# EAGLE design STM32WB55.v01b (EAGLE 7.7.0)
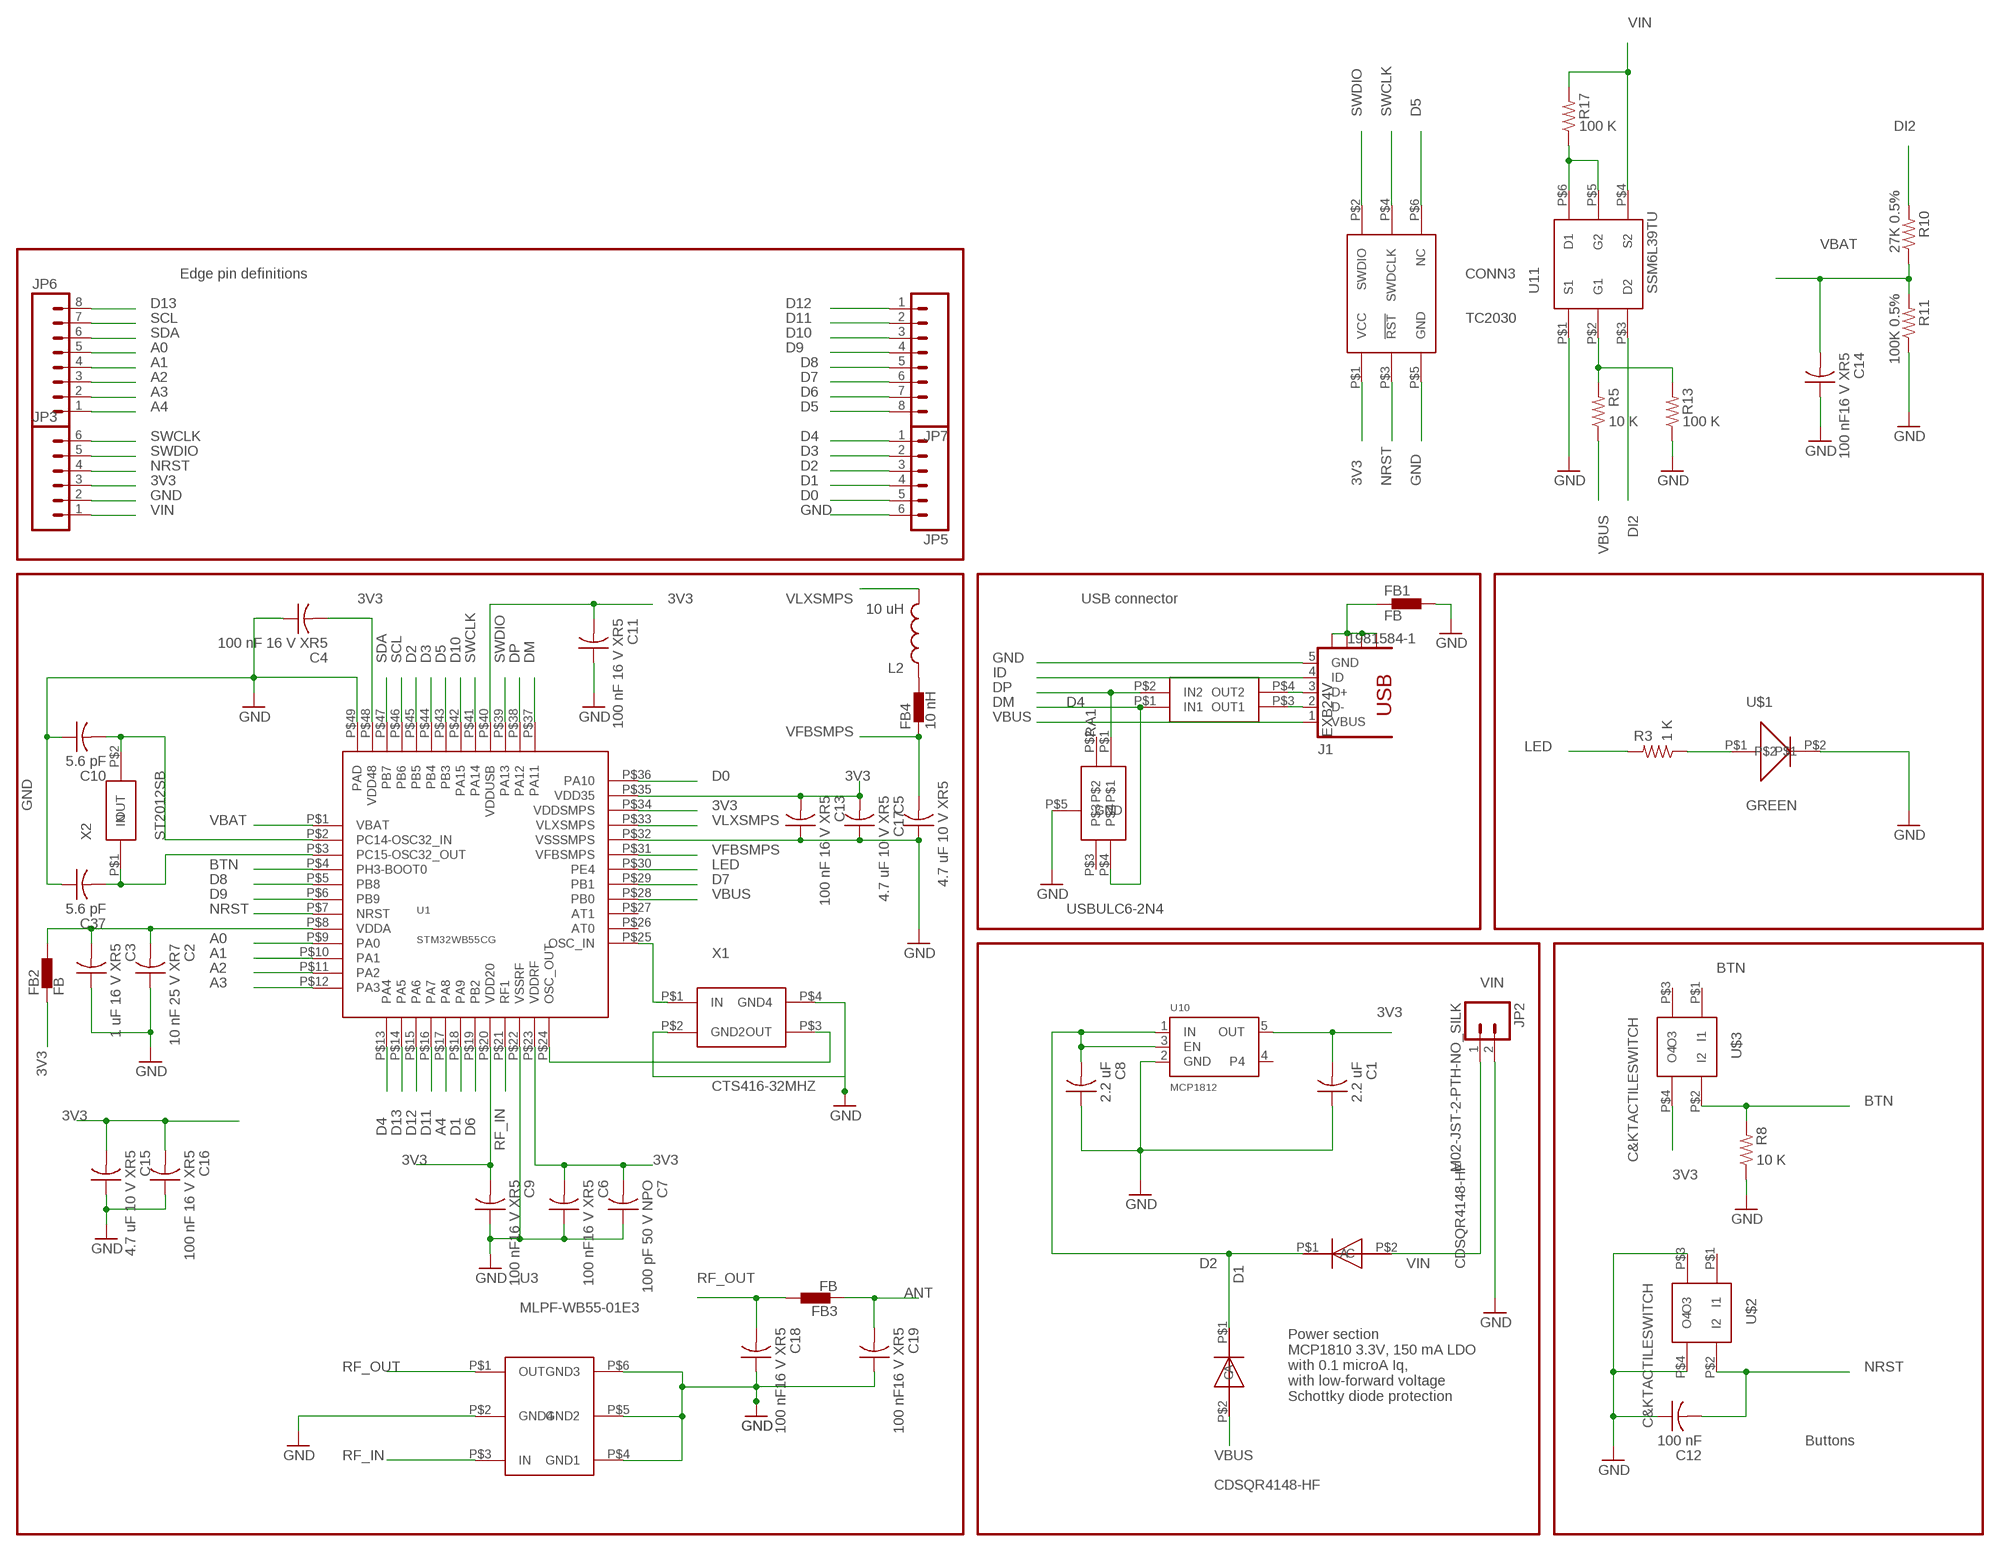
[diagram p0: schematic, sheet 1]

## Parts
C1  2.2 uF  C-US  [C0402_B]
C2  10 nF 25 V XR7  C-US  [C0402_B]
C3  1 uF 16 V XR5  C-US  [C0402_B]
C4  100 nF 16 V XR5  C-US  [C0402_B]
C5  4.7 uF 10 V XR5  C-US  [C0402_B]
C6  100 nF16 V XR5  C-US  [C0402_B]
C7  100 pF 50 V NPO  C-US  [C0402_B]
C8  2.2 uF  C-US  [C0402_B]
C9  100 nF16 V XR5  C-US  [C0402_B]
C10  5.6 pF  C-US  [C0402_B]
C11  100 nF 16 V XR5  C-US  [C0402_B]
C12  100 nF  C-US  [C0402_B]
C13  100 nF 16 V XR5  C-US  [C0402_B]
C14  100 nF16 V XR5  C-US  [C0402_B]
C15  4.7 uF 10 V XR5  C-US  [C0402_B]
C16  100 nF 16 V XR5  C-US  [C0402_B]
C17  4.7 uF 10 V XR5  C-US  [C0402_B]
C18  100 nF16 V XR5  C-US  [C0402_B]
C19  100 nF16 V XR5  C-US  [C0402_B]
C37  5.6 pF  C-US  [C0402_B]
CONN3  TC2030  [TC2030]
D1  CDSQR4148-HF  [CDSQR4148-HF]
D2  CDSQR4148-HF  [CDSQR4148-HF]
D4  USBULC6-2N4  [USBULC6-2N4]
FB1  FB  BLM15H  [0402]
FB2  FB  BLM15H  [0402]
FB3  FB  BLM15H  [0402]
FB4  10 nH  BLM15H  [0402]
J1  1981584-1  [1981584-1]
JP2  M02-JST-2-PTH-NO_SILK  [JST-2-PTH-NS]
JP3  M06NO_SILK  [1X06_NO_SILK]
JP5  M06NO_SILK  [1X06_NO_SILK]
JP6  M08NO_SILK  [1X08_NO_SILK]
JP7  M08NO_SILK  [1X08_NO_SILK]
L2  10 uH  INDUCTOR0805  [0805]
R3  1 K  R-US_  [R0402_B]
R5  10 K  R-US_  [R0402_B]
R8  10 K  R-US_  [R0402_B]
R10  27K 0.5%  R-US_  [R0402_B]
R11  100K 0.5%  R-US_  [R0402_B]
R13  100 K  R-US_  [R0402_B]
R17  100 K  R-US_  [R0402_B]
RA1  EXB24V  [EXB24V]
U1  STM32WB55CG  [ST32WB55CG]
U3  MLPF-WB55-01E3  [MLPF-WB55-01E3]
U10  MCP1812  VREG_SOT23-5  [SOT23-5]
U11  SSM6L39TU  [SSM6L39TU]
U$1  GREEN  0402LED  [0402LED]
U$2  C&KTACTILESWITCH  [C&KTACTILESWITCH]
U$3  C&KTACTILESWITCH  [C&KTACTILESWITCH]
X1  CTS416-32MHZ  [CTS416-32MHZ]
X2  ST2012SB  [ST2012SB]

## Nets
3V3: C1.2 C4.2 C5.2 C6.2 C7.2 C9.2 C11.2 C13.2 C15.2 C16.2 CONN3.P$1(VCC) FB2.1 JP3.3 U1.P$20(VDD20) U1.P$23(VDDRF) U1.P$34(VDDSMPS) U1.P$35(VDD35) U1.P$40(VDDUSB) U1.P$48(VDD48) U10.5(OUT) U$3.P$4(O4)
A0: JP6.5 U1.P$9(PA0)
A1: JP6.4 U1.P$10(PA1)
A2: JP6.3 U1.P$11(PA2)
A3: JP6.2 U1.P$12(PA3)
A4: JP6.1 U1.P$17(PA8)
ANT: C19.2 FB3.1
BTN: R8.2 U1.P$4(PH3-BOOT0) U$3.P$2(I2)
D0: JP5.5 U1.P$36(PA10)
D1: JP5.4 U1.P$18(PA9)
D2: JP5.3 U1.P$45(PB5)
D3: JP5.2 U1.P$44(PB4)
D4: JP5.1 U1.P$13(PA4)
D5: CONN3.P$6(NC) JP7.8 U1.P$43(PB3)
D6: JP7.7 U1.P$19(PB2)
D7: JP7.6 U1.P$29(PB1)
D8: JP7.5 U1.P$5(PB8)
D9: JP7.4 U1.P$6(PB9)
D10: JP7.3 U1.P$42(PA15)
D11: JP7.2 U1.P$16(PA7)
D12: JP7.1 U1.P$15(PA6)
D13: JP6.8 U1.P$14(PA5)
DI2: R10.2 U11.P$3(D2)
DM: D4.P$4 RA1.P$1(IN1) U1.P$37(PA11)
DP: D4.P$1 RA1.P$2(IN2) U1.P$38(PA12)
GND: C1.1 C2.1 C3.1 C4.1 C5.1 C6.1 C7.1 C8.1 C9.1 C10.1 C11.1 C12.1 C13.1 C14.1 C15.1 C16.1 C17.1 C18.1 C19.1 C37.1 CONN3.P$5(GND) D4.P$5(GND) FB1.2 J1.5(GND) JP2.2 JP3.2 JP5.6 R8.1 R11.1 R13.1 U1.P$22(VSSRF) U1.P$32(VSSSMPS) U1.P$49(PAD) U3.P$2(GND4) U3.P$4(GND1) U3.P$5(GND2) U3.P$6(GND3) U10.2(GND) U11.P$1(S1) U$1.P$2 U$2.P$3(O3) U$2.P$4(O4) X1.P$2(GND2) X1.P$4(GND4)
ID: J1.4(ID)
LED: R3.2 U1.P$30(PE4)
N$1: R3.1 U$1.P$1
N$2: C2.2 C3.2 FB2.2 U1.P$8(VDDA)
N$3: U1.P$25(OSC_IN) X1.P$1(IN)
N$4: U1.P$24(OSC_OUT) X1.P$3(OUT)
N$5: FB4.2 L2.1
N$7: C10.2 U1.P$2(PC14-OSC32_IN) X2.P$2(OUT)
N$8: C37.2 U1.P$3(PC15-OSC32_OUT) X2.P$1(IN)
N$12: R5.2 R13.2 U11.P$2(G1)
N$13: R17.1 U11.P$5(G2) U11.P$6(D1)
N$31: J1.3(D+) RA1.P$4(OUT2)
N$33: J1.2(D-) RA1.P$3(OUT1)
NRST: C12.2 CONN3.P$3(!RST) JP3.4 U1.P$7(NRST) U$2.P$2(I2)
PWRIN: C8.2 D1.P$1(C) D2.P$1(C) U10.1(IN) U10.3(EN)
RF_IN: U1.P$21(RF1) U3.P$3(IN)
RF_OUT: C18.2 FB3.2 U3.P$1(OUT)
SCL: JP6.7 U1.P$46(PB6)
SDA: JP6.6 U1.P$47(PB7)
SWCLK: CONN3.P$4(SWDCLK) JP3.6 U1.P$41(PA14)
SWDIO: CONN3.P$2(SWDIO) JP3.5 U1.P$39(PA13)
USB_SHIELD: FB1.1 J1.S1 J1.S2 J1.S3 J1.S4
VBAT: C14.2 R10.1 R11.2 U1.P$1(VBAT)
VBUS: D2.P$2(A) J1.1(VBUS) R5.1 U1.P$28(PB0)
VFBSMPS: C17.2 FB4.1 U1.P$31(VFBSMPS)
VIN: D1.P$2(A) JP2.1 JP3.1 R17.2 U11.P$4(S2)
VLXSMPS: L2.2 U1.P$33(VLXSMPS)
Unconnected: D4.P$2 D4.P$3 U1.P$26(AT0) U1.P$27(AT1) U10.4 U$2.P$1(I1) U$3.P$1(I1) U$3.P$3(O3)

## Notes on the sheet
- Edge pin definitions
- USB connector
- Power section
  MCP1810 3.3V, 150 mA LDO
  with 0.1 microA Iq, 
  with low-forward voltage 
  Schottky diode protection
- Buttons

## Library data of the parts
C1-C19 C37 = Spark:C-US: Capacitor
CONN3 = Kris:TC2030: TC2030 SWD pogo pin contact pad
D1 D2 = Kris:CDSQR4148-HF: ComChip's CDSQR4148-HF high speed 150 mA Io diode
D4 = Kris:USBULC6-2N4: ST TVS diode ESD Protection USBULC6-2N4
FB1-FB4 = STM32L433SARA.AssetTracker.v01:BLM15H: EMIFIL (R) Chip Ferrite Bead for GHz Noise
J1 = con-usb:1981584-1: Receptacle, micro-USB, type A/B Tyco Electronics; MF: Hirose; MPN: ZX62-AB-5PA(11)
JP2 = SparkFun-Connectors:M02: Standard 2-pin 0.1" header. Use with
JP3 JP5 = SparkFun-Connectors:M06: Header 6 Standard 6-pin 0.1" header. Use with straight break away headers (SKU : PRT-00116), right angle break away headers (PRT-00553), swiss pins (PRT-00743), machine pins (PRT-00117), and female headers (PRT-00115). Molex polarized connector foot print use with SKU : PRT-08094 with associated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
JP6 JP7 = SparkFun-Connectors:M08: Header 8 Standard 8-pin 0.1" header. Use with straight break away headers (SKU : PRT-00116), right angle break away headers (PRT-00553), swiss pins (PRT-00743), machine pins (PRT-00117), and female headers (PRT-00115).
L2 = SparkFun-Passives:INDUCTOR: Inductors
R3 R5 R8 R10 R11 R13 R17 = Spark:R-US_: 0402 Resistor
RA1 = Kris:EXB24V: Panasonic EXB24 22 Ohm series resistor pair
U1 = Kris:STM32WB55CG: STM32WB55CG 7 mm x 7 mm UFQFPN48 https://www.st.com/en/microcontrollers/stm32wbx5.html?querycriteria=productId=LN2047
U3 = Kris:MLPF-WB55-01E3: MLPF-WB55-01E3
U10 = ModernDevice:VREG_SOT23-5: SOT23-5 Fixed Voltage Regulators To better organise some of the SOT23-5 fixed voltage regulators in this library, this new part was created. Part Current Out V Out V In V Dropout Digikey Part No. ADP121 150mA 3.3V 3.4-5.5V 0.09V @ 150mA ADP121-AUJZ33R7CT-ND ADP121 150mA 3.0V 3.1-5.5V 0.09V @ 150mA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
U11 = Kris:SSM6L39TU: SSM6L39TU Dual Mosfet https://www.mouser.com/datasheet/2/408/SSM6L39TU_datasheet_en_20140301-771389.pdf
U$1 = Kris:0402LED: 0402led
U$2 U$3 = Kris:C&KTACTILESWITCH: C&K Tactile Switch 611-PTS810SJS250SMTR
X1 = Kris:CTS416-32MHZ: 32 MHz CTS416 crystal
X2 = Kris:ST2012SB: Kyocera 2.0 x 1.2 mm 32.768 20kHz ppm 4 pf crystal

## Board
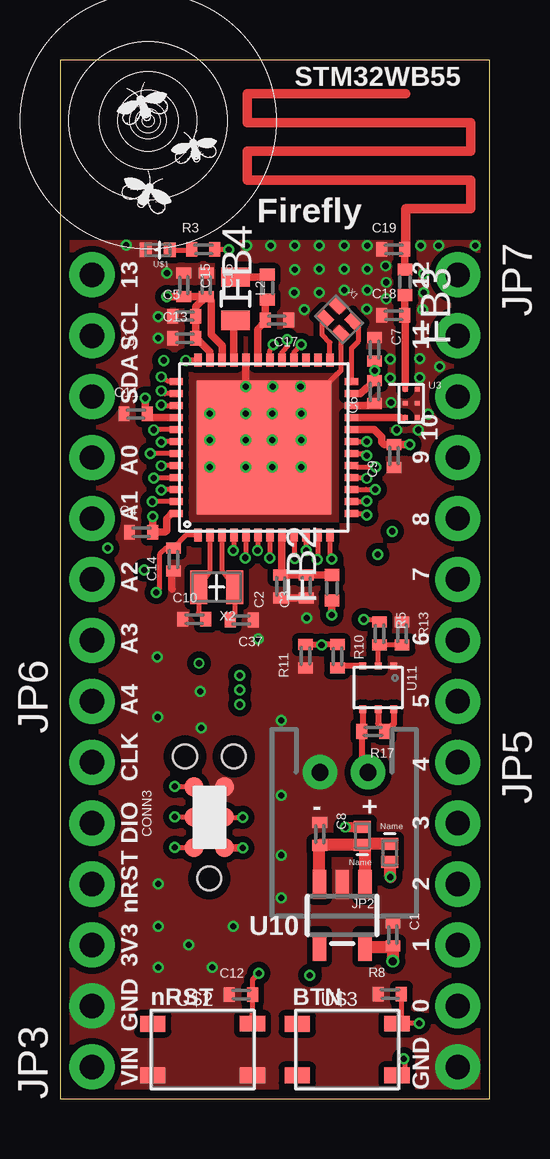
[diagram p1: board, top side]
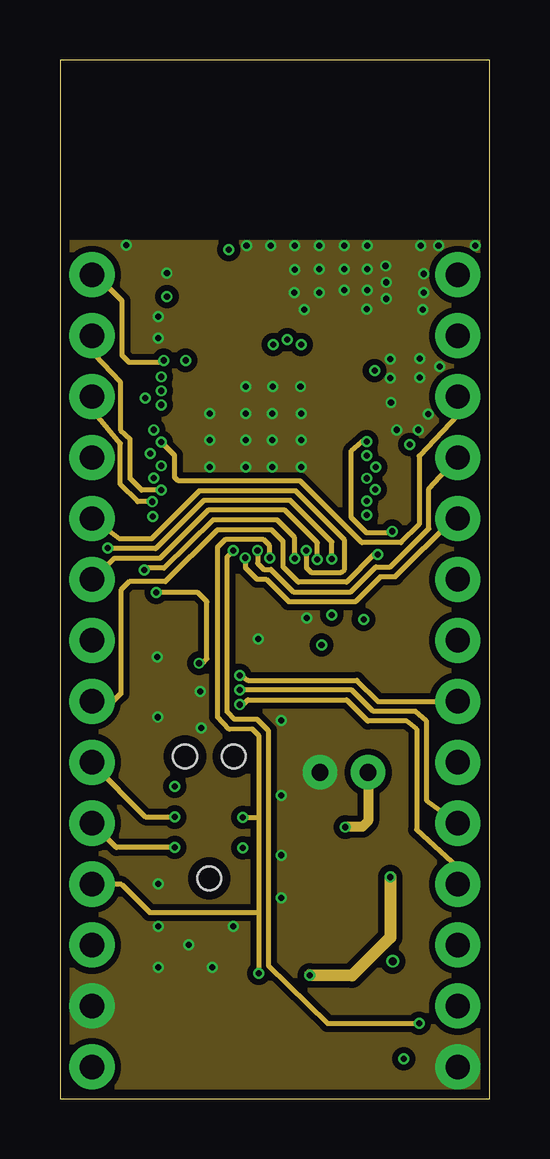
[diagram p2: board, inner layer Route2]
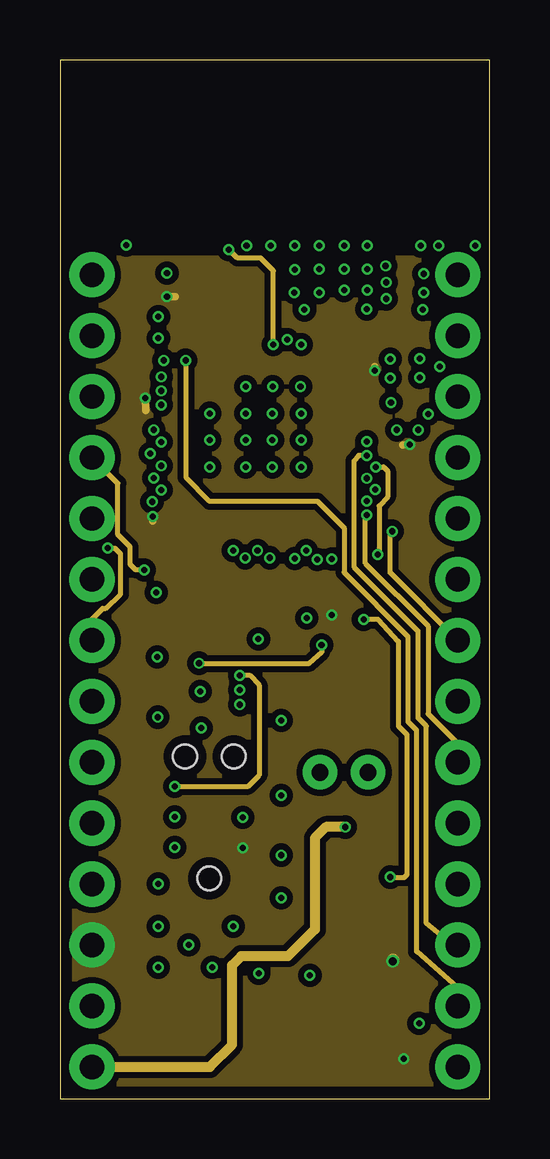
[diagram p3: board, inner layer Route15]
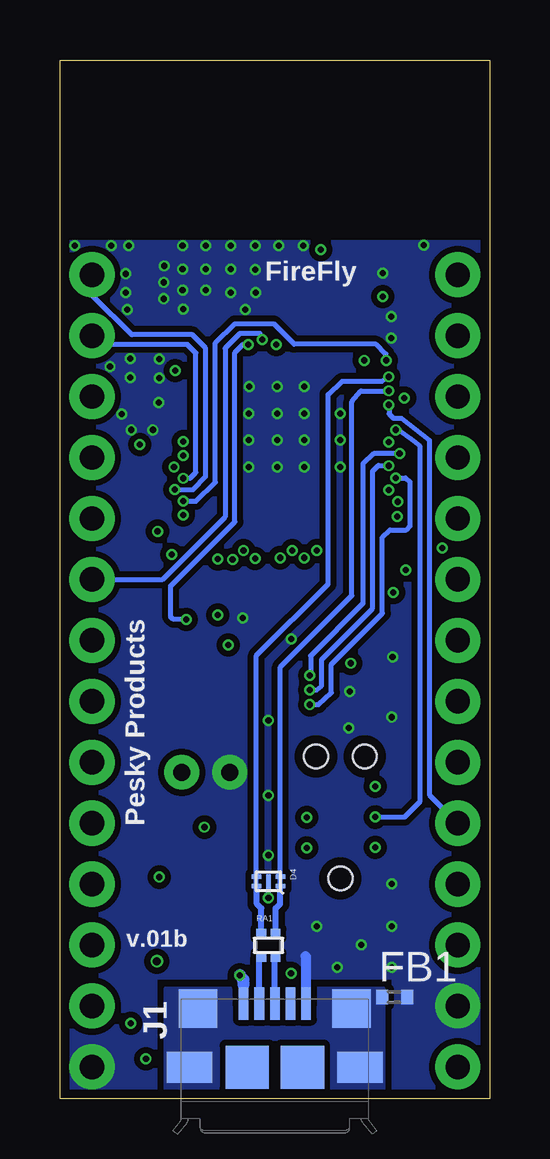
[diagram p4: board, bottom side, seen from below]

Size 17.91 x 43.31 mm. Coordinates in mm from the lower left corner, seen from the top.
Outline: 0,0 17.91,0 17.91,43.31 0,43.31 0,0
Copper layers (1*2*15*16): Top 0.035559375mm / dielectric 0.17018125mm / Route2 0.01778125mm / dielectric 47mil / Route15 0.01778125mm / dielectric 0.17018125mm / Bottom 0.035559375mm
Design rules "OSHPark-4layer *": minimum track width 5mil, minimum drill 10mil, track to track 5mil, track to pad 5mil, pad to pad 5mil, via to via 5mil, smd to smd 5mil, copper to edge 15mil, drill to drill 6mil, minimum pad ring 4mil, minimum via ring 4mil, stop-mask expansion 4mil, vias tented up to drill 20mil, thermal gap 10mil

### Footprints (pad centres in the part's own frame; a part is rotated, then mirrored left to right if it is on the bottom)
C0402_B = smd 0.457 x 0.61: 1 -0.483,0; 2 0.483,0
TC2030 = smd 0.787 x 0.787: P$1 -1.27,-0.635; P$2 -1.27,0.635; P$3 0,-0.635; P$4 0,0.635; P$5 1.27,-0.635; P$6 1.27,0.635 | hole 0.991: -2.54,0; 2.54,1.016; 2.54,-1.016
CDSQR4148-HF = smd 0.7 x 0.5: P$1 0,0.375; P$2 0,-0.375
USBULC6-2N4 = smd 0.2 x 0.4: P$1 0.2,0.5; P$2 -0.2,0.5; P$3 -0.2,-0.5; P$4 0.2,-0.5 | smd 0.6 x 0.2: P$5 0,0
0402 = smd 0.5 x 0.61: 1 -0.5,0; 2 0.55,0
1981584-1 = smd 0.4 x 1.35: 1 -1.3,4.1; 2 -0.65,4.1; 3 0,4.1; 4 0.65,4.1; 5 1.3,4.1 | smd 1.8 x 1.8: M1 -1.15,1.45; M2 1.15,1.45 | smd 1.9 x 1.3: S1 -3.55,1.45; S2 3.55,1.45 | smd 1.6 x 1.6: S3 -3.2,3.885; S4 3.2,3.885
JST-2-PTH-NS = drill 0.7 pad 1.448: 1 -1,0; 2 1,0
1X06_NO_SILK = drill 1.016 pad 1.88: 1 0,0; 2 2.54,0; 3 5.08,0; 4 7.62,0; 5 10.16,0; 6 12.7,0
1X08_NO_SILK = drill 1.016 pad 1.88: 1 0,0; 2 2.54,0; 3 5.08,0; 4 7.62,0; 5 10.16,0; 6 12.7,0; 7 15.24,0; 8 17.78,0
0805 = smd 0.8 x 1.2: 1 -0.9,0; 2 0.9,0
R0402_B = smd 0.457 x 0.61: 1 -0.483,0; 2 0.483,0
EXB24V = smd 0.4 x 0.36: P$1 -0.3,0.5; P$2 0.3,0.5; P$3 -0.3,-0.5; P$4 0.3,-0.5
ST32WB55CG = smd 0.55 x 0.3: P$1 -3.65,2.75; P$2 -3.65,2.25; P$3 -3.65,1.75; P$4 -3.65,1.25; P$5 -3.65,0.75; P$6 -3.65,0.25; P$7 -3.65,-0.25; P$8 -3.65,-0.75; P$9 -3.65,-1.25; P$10 -3.65,-1.75; P$11 -3.65,-2.25; P$12 -3.65,-2.75; P$25 3.65,-2.75; P$26 3.65,-2.25; P$27 3.65,-1.75; P$28 3.65,-1.25; P$29 3.65,-0.75; P$30 3.65,-0.25; P$31 3.65,0.25; P$32 3.65,0.75; P$33 3.65,1.25; P$34 3.65,1.75; P$35 3.65,2.25; P$36 3.65,2.75 | smd 0.3 x 0.55: P$13 -2.75,-3.65; P$14 -2.25,-3.65; P$15 -1.75,-3.65; P$16 -1.25,-3.65; P$17 -0.75,-3.65; P$18 -0.25,-3.65; P$19 0.25,-3.65; P$20 0.75,-3.65; P$21 1.25,-3.65; P$22 1.75,-3.65; P$23 2.25,-3.65; P$24 2.75,-3.65; P$37 2.75,3.65; P$38 2.25,3.65; P$39 1.75,3.65; P$40 1.25,3.65; P$41 0.75,3.65; P$42 0.25,3.65; P$43 -0.25,3.65; P$44 -0.75,3.65; P$45 -1.25,3.65; P$46 -1.75,3.65; P$47 -2.25,3.65; P$48 -2.75,3.65 | smd 5.6 x 5.6: P$49 0,0
MLPF-WB55-01E3 = smd 0.2 x 0.2: P$1 -0.25,0.587; P$2 -0.25,0; P$3 -0.25,-0.587; P$4 0.25,-0.587; P$5 0.25,0; P$6 0.25,0.587
SOT23-5 = smd 0.55 x 1.2: 1 -0.95,-1.3; 2 0,-1.3; 3 0.95,-1.3; 4 0.95,1.3; 5 -0.95,1.3
SSM6L39TU = smd 0.3 x 0.3: P$1 -0.9,0.65; P$2 -0.9,0; P$3 -0.9,-0.65; P$4 0.9,-0.65; P$5 0.9,0; P$6 0.9,0.65
0402LED = smd 0.5 x 0.6: P$1 -0.5,0; P$2 0.5,0
C&KTACTILESWITCH = smd 1.05 x 0.65: P$1 -2.075,1.073; P$2 2.075,1.075; P$3 -2.075,-1.075; P$4 2.075,-1.075
CTS416-32MHZ = smd 0.67 x 0.48: P$1 -0.485,-0.38; P$2 0.485,-0.38; P$3 0.485,0.38; P$4 -0.485,0.38
ST2012SB = smd 0.7 x 1.4: P$1 -0.75,0; P$2 0.75,0

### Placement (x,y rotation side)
C1  13.87,6.86 270 top
C2  9.19,21.36 90 top
C3  10.26,21.36 90 top
C4  3.38,23.62 0 top
C5  5.18,32.63 0 top
C6  13.11,29.46 90 top
C7  13.11,31.24 270 top
C8  10.82,11.05 270 top
C9  13.92,26.8 90 top
C10  5.59,19.99 0 top
C11  3.15,28.55 0 top
C12  7.54,4.34 0 top
C13  5.18,31.7 0 top
C14  4.72,22.48 90 top
C15  5.16,33.93 270 top
C16  6.1,33.93 270 top
C17  9.04,32.46 180 top
C18  13.89,32.66 0 top
C19  13.89,35.41 0 top
C37  7.57,19.96 180 top
CONN3  6.22,11.73 90 top
D1  12.6,10.97 180 top
D2  13.74,10.26 0 top
D4  9.22,9.07 270 bottom
FB1  3.99,4.24 0 bottom
FB2  11.33,21.29 90 top
FB3  14.37,34.06 270 top
FB4  8.64,33.81 90 top
J1  8.95,-0.13 0 bottom
JP2  11.84,13.61 180 top
JP3  1.33,1.33 90 top
JP5  16.57,14.03 270 top
JP6  1.33,16.57 90 top
JP7  16.57,34.35 270 top
L2  7.32,33.35 270 top
R3  5.97,35.41 0 top
R5  13.31,19.41 270 top
R8  13.74,4.37 0 top
R10  11.56,18.45 270 top
R11  10.22,18.45 90 top
R13  14.25,19.41 270 top
R17  13.06,15.32 180 top
RA1  9.22,6.4 0 bottom
U1  8.5,27.15 90 top
U3  14.63,28.99 0 top
U10  11.76,7.65 180 top
U11  13.26,17.14 270 top
U$1  4.06,35.38 180 top
U$2  5.94,2.06 0 top
U$3  11.96,2.06 0 top
X1  11.63,32.49 315 top
X2  6.53,21.34 180 top

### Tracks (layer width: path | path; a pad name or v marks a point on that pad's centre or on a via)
3V3  (via drill 0.25, 0.33)
  Top 0.203: U$3.P$4 14.38,1.22 14.38,1.63 v14.33,1.68
  Top 0.305: U1.P$35 6.25,31.14 5.69,31.7 5.69,31.67 C13.2 C5.2 5.66,33.03 C16.2 | U1.P$40 3.62,28.4 3.68,28.42 3.68,28.43 | C7.2 v13.11,30.35 C6.2 12.51,29.4 U1.P$23 | v3.86,24.28 C4.2 4.37,23.62 4.45,23.7 4.45,24.18 4.64,24.4 U1.P$48 | v14.58,27.28 C9.2 13.51,27.28 13.41,27.38 13.41,27.58 13.09,27.9 U1.P$20 | 3.68,28.43 C11.2 3.56,28.7 v3.56,29.21 | 3.68,28.43 3.68,28.46 | 11.37,20.84 FB2.1 v11.33,20.17 | C16.2 6.12,33.4 6.3,33.27 6.3,31.85 6.76,31.39 6.76,30.81 U1.P$34 | C16.2 C15.2 4.45,33.45 v4.46,33.44 | CONN3.P$1 v7.62,10.46
  Top 0.508: U10.5 13.86,6.34 | 13.86,6.34 C1.2 | 13.86,6.34 13.86,5.77 v13.87,5.74
  Route15 0.203: v14.33,1.68 14.33,1.63 14.38,1.57
  Route15 0.305: v3.56,29.21 3.58,28.69 | v13.11,30.35 13.11,30.53 | v3.86,24.28 3.86,24.08 | v14.58,27.28 14.28,27.25 | v4.46,33.44 4.8,33.44 | v11.33,20.17 11.33,20.24
  Route15 0.508: v13.87,5.74 13.89,5.79 13.87,5.82
  pour Route15 (isolate 0.254, no thermals): 0.64,35.05 17.27,35.05 17.27,0.64 0.64,0.64
A0  (via drill 0.25)
  Top 0.203: v9.78,22.53 9.78,23.41 U1.P$9
  Route2 0.203: v9.78,22.53 9.78,23.39 9.04,24.13 6.38,24.13 4.34,22.12 3.5,22.12 v3.5,22.05
  Route15 0.203: v3.5,22.05 3.15,22.05 2.92,22.28 2.92,23.01 2.41,23.52 2.41,25.65 JP6.5
A1  (via drill 0.25)
  Top 0.203: U1.P$10 10.25,22.88 v10.26,22.86
  Route2 0.203: JP6.4 2.49,23.34 3.81,23.34 5.82,25.35 9.8,25.35 11.86,23.29 11.86,22.07 11.71,21.95 10.46,21.95 10.26,22.15 v10.26,22.86
A2  (via drill 0.25)
  Top 0.203: U1.P$11 10.75,22.58 v10.72,22.48
  Route2 0.203: v10.72,22.48 10.72,23.19 9.37,24.54 6.17,24.54 4.17,22.53 2.26,22.53 JP6.3
A3  (via drill 0.25)
  Top 0.203: U1.P$12 11.25,22.69 v11.33,22.5
  Route2 0.203: v11.33,22.5 11.33,23.22 9.6,24.94 5.99,24.94 3.99,22.94 2.08,22.94 v1.98,22.96
  Route15 0.203: v1.98,22.96 2.29,22.96 2.52,22.73 2.52,21.03 1.91,20.45 1.78,20.45 1.33,20 JP6.2
A4  (via drill 0.25)
  Top 0.203: U1.P$17 12.33,26.4 12.37,26.34 v13.16,26.34
  Route2 0.203: JP6.1 1.35,16.59 2.21,16.59 2.54,16.89 2.54,21.21 2.9,21.57 4.39,21.57 6.55,23.72 8.81,23.72 9.3,23.24 9.3,22.17 9.93,21.54 11.94,21.54 13.08,22.68 v13.25,22.7
  Route15 0.203: v13.16,26.34 13.49,26.34 13.65,26.18 13.65,25.09 13.3,24.71 13.3,22.75 v13.25,22.7
ANT
  Top 0.305: FB3.1 C19.2 14.38,35.41 14.41,35.43
  Top 0.4: 14.41,35.43 14.41,37.1 17.11,37.1 17.11,38.3 7.81,38.3 7.81,39.5 17.11,39.5 17.11,40.7 7.81,40.7 7.81,41.9 14.41,41.9
BTN  (via drill 0.25)
  Top 0.203: U1.P$4 7.25,22.94 v7.21,22.86 | v14.96,3.15 13.98,3.15 U$3.P$2 14.22,3.39 R8.2
  Route2 0.203: v14.96,3.15 11.15,3.15 8.69,5.56 8.69,15.35 8.22,15.82 7.28,15.82 6.96,16.14 6.96,22.58 v7.21,22.86
D0  (via drill 0.25)
  Top 0.203: U1.P$36 5.33,30.8 v5.23,30.79
  Route15 0.203: JP5.5 16.57,4.64 14.86,6.15 14.86,15.37 14.5,15.72 14.5,19.25 11.84,21.95 11.84,23.8 10.72,24.92 6.22,24.92 5.26,25.91 5.26,30.76 v5.23,30.79
D1  (via drill 0.25)
  Top 0.203: U1.P$18 12.62,26.9 v12.78,26.81
  Route15 0.203: JP5.4 16.34,6.41 15.27,7.32 15.27,15.54 14.91,15.9 14.91,19.51 12.24,22.17 12.24,26.59 12.45,26.82 v12.78,26.81
D2  (via drill 0.25)
  Top 0.203: U1.P$45 4.7,25.9 4.67,25.93 4.7,25.93 4.62,25.88 v3.91,25.88
  Route2 0.203: JP5.3 16.59,8.97 16.59,9.65 14.86,11.23 14.86,15.42 14.45,15.75 12.83,15.75 11.94,16.64 7.82,16.64 7.64,16.43 v7.49,16.43
  Bottom 0.203: v3.91,25.88 3.5,25.88 3.33,25.73 3.33,23.88 3.48,23.72 4.17,23.72 4.47,23.42 4.47,20.24 6.6,18.11 6.6,16.94 7.14,16.43 v7.49,16.43
D3  (via drill 0.25)
  Top 0.203: U1.P$44 4.25,26.4 v4.22,26.39
  Route2 0.203: v7.49,17.04 12.17,17.04 13.06,16.15 14.81,16.15 15.27,15.75 15.27,12.45 JP5.2
  Bottom 0.203: v4.22,26.39 4.31,26.4 4.64,26.4 4.88,26.17 4.88,20.45 7.01,18.31 7.01,17.22 7.21,17.04 v7.49,17.04
D4  (via drill 0.25)
  Top 0.203: U1.P$13 12.68,24.4 v12.78,24.33
  Route15 0.203: v12.78,24.33 12.72,24.16 12.72,22.33 15.34,19.71 15.34,16.05 16.57,14.82 JP5.1
D5  (via drill 0.25)
  Top 0.203: U1.P$43 v3.76,26.9 | CONN3.P$6 4.78,13.01 v4.78,13.03
  Route2 0.203: JP7.8 13.26,16.56 12.37,17.45 7.82,17.45 7.57,17.65 v7.49,17.65
  Route15 0.203: 7.48,17.67 7.52,17.67 | 7.52,17.67 7.9,17.67 8.29,17.25 8.29,13.49 7.84,13.03 v4.78,13.03 | v7.49,17.65 7.51,17.65 7.52,17.67
  Bottom 0.203: v3.76,26.9 4.83,26.9 5.28,26.47 5.28,20.65 7.47,18.47 7.47,17.7 v7.49,17.65
D6  (via drill 0.25)
  Top 0.203: U1.P$19 12.72,27.4 v12.78,27.39
  Route2 0.203: v13.84,23.66 13.6,23.6 12.78,23.6 12.14,24.23 12.14,27.03 12.57,27.41 12.76,27.41 v12.78,27.39
  Route15 0.203: JP7.7 13.75,21.93 13.75,23.66 v13.84,23.66
D7  (via drill 0.25)
  Top 0.203: U1.P$29 9.25,31.09 9.47,31.37 v9.47,31.65
  Bottom 0.203: v9.47,31.65 9.47,31.77 9.58,31.9 10.41,31.9 11.02,31.29 11.02,24.26 13.63,21.65 JP7.6
D8  (via drill 0.25)
  Top 0.203: U1.P$5 7.75,22.61 v7.72,22.55
  Route2 0.203: v7.72,22.55 7.72,22.15 8.2,21.67 8.59,21.67 9.53,20.73 12.32,20.73 13.36,21.77 13.97,21.77 16.38,24.18 JP7.5
D9  (via drill 0.25)
  Top 0.203: U1.P$6 8.25,22.98 v8.23,22.86
  Route2 0.203: JP7.4 15.37,25.43 15.37,23.77 13.77,22.17 13.16,22.17 12.12,21.13 9.73,21.13 8.79,22.07 8.48,22.07 8.23,22.33 v8.23,22.86
D10  (via drill 0.25)
  Top 0.203: U1.P$42 4.42,27.4 v4.22,27.38
  Route2 0.203: JP7.3 16.57,28.51 14.96,26.8 14.96,23.95 14.2,23.19 12.57,23.19 10.01,25.76 4.93,25.76 4.78,25.91 4.78,26.82 v4.22,27.38
D11  (via drill 0.25)
  Top 0.203: U1.P$16 12.71,25.9 v12.78,25.87
  Bottom 0.203: v12.78,25.87 12.48,25.87 12.24,26.11 12.24,31.09 12.6,31.45 16.15,31.45 JP7.2
D12  (via drill 0.25)
  Top 0.203: U1.P$15 12.75,25.4 v13.13,25.4
  Bottom 0.203: v13.13,25.4 12.36,25.4 11.84,25.93 11.84,31.29 12.39,31.85 14.91,31.85 16.57,33.49 JP7.1
D13  (via drill 0.25)
  Top 0.203: U1.P$14 12.66,24.9 v12.78,24.92
  Route2 0.203: JP6.8 1.5,34.35 2.58,33.27 2.58,31 2.87,30.71 4.24,30.71 v4.32,30.79
  Bottom 0.203: v12.78,24.92 12.24,24.92 11.43,25.7 11.43,31.52 10.62,32.31 9,32.31 8.15,31.46 4.74,31.46 4.33,31.05 4.33,30.79 v4.32,30.79
DI2
  Top 0.254: U11.P$3 11.63,18.05 R10.2
DM  (via drill 0.25)
  Top 0.203: U1.P$37 4.51,29.9 v4.22,30.1
  Bottom 0.203: D4.P$4 9.72,18.47 6.73,21.46 6.73,29.36 6.15,29.92 4.48,29.92 v4.22,30.1
  Bottom 0.254: RA1.P$1 9.52,7.95 9.7,8.13 9.7,8.85 D4.P$4
DP  (via drill 0.25)
  Top 0.203: U1.P$38 4.37,29.4 v4.22,29.52
  Bottom 0.203: D4.P$1 8.72,18 5.74,20.98 5.74,29.06 5.37,29.52 v4.22,29.52
  Bottom 0.254: RA1.P$2 8.92,7.95 8.74,8.13 8.74,8.85 D4.P$1
GND  (via drill 0.25)
  Top 0.203: X1.P$2 11.71,30.35 v8.85,27.46
  Top 0.305: U1.P$32 7.75,29.95 7.75,30.02 | U1.P$22 13.08,28.9 C6.1 | C14.1 4.65,22.05 4.65,21.29 4.67,21.26 | C2.1 C3.1
  Bottom 0.203: D4.P$5 v9.22,8.38
  Bottom 0.406: J1.5 7.65,5.93 7.67,5.94
  other vias: 7.73,27.46 11.84,35.56 15.04,35.56 15.16,33.6 13.59,33.35 12.8,33.71 12.8,35.56 15.11,32.89 13.77,30.84 14.99,30.86 14.99,30.07 13.77,30.05 13.79,29.03 9.22,10.16 9.22,12.65 6.24,28.57 8.85,26.34 7.73,29.69 8.85,28.57 7.73,28.57 7.73,26.34 6.24,26.34 6.24,27.46 12.78,32.92 2.76,35.59 4.46,34.42 4.1,32.6 15.34,28.55 15.82,30.53 14.94,27.89 10.79,35.56 9.78,35.56 8.79,35.56 7.77,35.56 11.84,34.59 10.79,34.59 11.84,33.71 17.3,35.56 15.77,35.56 15.16,34.39 10.05,28.57 10.05,27.46 10.05,26.34 8.27,19.18 9.22,15.77 10.29,20.05 4.1,31.71 9.78,34.57 10.79,33.6 9.75,33.6 10.19,32.89 14.03,27.89 4.05,18.43 4.08,15.91 5.84,16.98 5.88,15.46 10.02,29.69 8.86,29.69 13.56,34.72 12.8,34.59 13.59,34.04 4.09,7.19 6.35,5.49 7.21,7.19 4.09,5.49 5.36,6.43 4.09,8.97
  pour Route2 (isolate 0.254, no thermals): 0,35.69 17.91,35.69 17.91,0 0,0
  pour Top (isolate 0.254, no thermals): 0,35.69 17.91,35.69 17.91,0 0,0
  pour Bottom (isolate 0.254, no thermals): 13.97,0 17.91,0 17.91,35.69 0,35.69 0,0 3.96,0 3.96,5.08 13.97,5.08
LED  (via drill 0.25)
  Top 0.203: U1.P$30 8.75,31.2 v8.89,31.45 | v7.04,35.41 R3.2
  Route15 0.203: v8.89,31.45 8.89,34.52 8.36,35.05 7.39,35.05 v7.04,35.41
N$1
  Top 0.203: U$1.P$1 5.46,35.38 R3.1
N$2
  Top 0.305: U1.P$8 9.25,21.95 C2.2 C3.2 FB2.2
N$3
  Top 0.203: U1.P$25 11.25,31.53 10.92,31.85 10.92,32.54 X1.P$1
N$4
  Top 0.203: U1.P$24 12.15,31.3 12.45,31.6 12.45,32.29 X1.P$3
N$5
  Top 0.305: L2.1 8.52,34.25 FB4.2
N$7
  Top 0.203: U1.P$2 6.25,21.96 X2.P$2 5.78,20.28 C10.2
N$8
  Top 0.203: U1.P$3 6.75,22.02 X2.P$1 7.28,20.21 C37.2
N$12
  Top 0.203: R13.2 R5.2 13.26,19 U11.P$2
N$13
  Top 0.254: U11.P$5 13.26,15.65 R17.1 13.91,15.64 U11.P$6
N$31
  Bottom 0.254: J1.3 8.95,5.87 RA1.P$4
N$33
  Bottom 0.254: J1.2 9.6,5.82 RA1.P$3
NRST  (via drill 0.25)
  Top 0.203: U$2.P$2 C12.2 8.03,4.98 v8.28,5.23 | U1.P$7 8.75,22.67 v8.74,22.55 | CONN3.P$3 v7.62,11.73
  Route2 0.203: v8.74,22.55 8.74,23.06 8.48,23.32 6.88,23.32 6.55,22.99 6.55,15.94 7.06,15.4 8.01,15.42 8.28,15.15 8.28,11.73 | 8.28,11.73 8.28,7.8 | 8.28,7.8 v8.28,5.23 8.27,5.22 | JP3.4 1.35,8.94 2.56,8.94 3.73,7.77 8.26,7.77 8.28,7.8 | v7.62,11.73 8.28,11.73
PWRIN
  Top 0.406: 12.97,10.64 D1.P$1 12.71,10.49 | 10.85,10.6 C8.2
  Top 0.508: D2.P$1 12.97,10.64 | D1.P$1 10.85,10.6 | U10.3 10.81,10.56 C8.2 | U10.1 12.71,10.49
RF_IN
  Top 0.203: U3.P$3
  Top 0.254: 14.18,28.4 U3.P$3
  Top 0.305: U1.P$21 14.18,28.4
RF_OUT
  Top 0.254: U3.P$1 14.38,29.57 14.38,29.77
  Top 0.305: 14.38,29.77 C18.2 FB3.2
SCL  (via drill 0.25)
  Top 0.203: U1.P$46 4.24,25.4 v4.22,25.38
  Route2 0.203: JP6.7 1.44,31.71 1.44,31.03 2.52,29.87 2.52,27.89 2.92,27.51 2.92,25.86 3.4,25.38 v4.22,25.38
SDA  (via drill 0.25)
  Top 0.203: U1.P$47 3.83,24.9 v3.83,24.89
  Route2 0.203: v3.83,24.89 3.23,24.89 2.52,25.61 2.52,27.33 1.52,28.52 1.52,29.09 JP6.6
SWCLK  (via drill 0.25)
  Top 0.203: 4.81,27.94 U1.P$41 4.08,27.9 v3.91,27.89 | CONN3.P$4 5.08,11.73 v4.78,11.75
  Route2 0.203: JP3.6 1.33,13.98 3.56,11.76 4.76,11.76 v4.78,11.75
  Bottom 0.203: v3.91,27.89 3.79,27.89 3.28,27.51 2.92,27.23 2.92,12.37 3.56,11.73 4.76,11.73 v4.78,11.75
SWDIO  (via drill 0.25)
  Top 0.203: v4.22,28.93 4.29,28.91 U1.P$39 | CONN3.P$2 5,10.46 v4.78,10.48
  Route2 0.203: v4.78,10.48 2.35,10.48 JP3.5
  Bottom 0.203: JP3.5 2.52,12.68 2.52,27.46 3.68,28.37 4.01,28.37 4.19,28.55 4.19,28.88 v4.22,28.93
USB_SHIELD
  pour Bottom (isolate 0.254, no thermals): 4.47,0 13.46,0 13.46,4.57 4.47,4.57
VBAT  (via drill 0.25)
  Top 0.203: U1.P$1 5.24,23.5 C14.2 4.42,22.96 4.14,22.68 4.14,21.26 v4.01,21.11
  Top 0.254: R11.2 10.88,18.94 v10.9,18.92 11.04,18.94 R10.1
  Route2 0.203: v5.79,18.16 5.94,18.16 6.12,18.34 6.12,20.73 5.74,21.11 v4.01,21.11
  Route15 0.203: v5.79,18.16 10.39,18.16 10.9,18.62 v10.9,18.92
VBUS  (via drill 0.25)
  Top 0.203: U1.P$28 9.75,31.11 v10.06,31.45 | v12.65,19.99 13.13,19.99 R5.1
  Top 0.406: 13.77,9.86 D2.P$2
  Top 0.508: v13.77,9.25 13.77,9.86
  Route2 0.508: v13.77,9.25 13.77,6.73 12.17,5.13 v10.41,5.16
  Route15 0.203: 13.72,9.3 v13.77,9.25 13.79,9.22 14.33,9.22 14.45,9.35 14.45,15.19 14.1,15.54 14.1,19.07 13.26,19.99 v12.65,19.99
  Bottom 0.203: v10.06,31.45 10.29,31.45 10.62,31.11 10.62,24.05 13.31,21.36 13.31,20.12 13.18,19.99 v12.65,19.99
  Bottom 0.406: J1.1 10.25,4.77
  Bottom 0.508: 10.25,4.77 10.26,4.98 v10.41,5.16
VFBSMPS
  Top 0.305: U1.P$31 8.25,32.07 C17.2 8.56,33.23 FB4.1
VIN  (via drill 0.25)
  Top 0.254: U11.P$4 12.61,15.33 R17.2 12.57,13.88 JP2.1
  Top 0.406: v11.89,11.33 12.41,11.33 D1.P$2
  Route2 0.406: JP2.1 12.84,11.59 D1.P$2 11.91,11.35 v11.89,11.33
  Route15 0.203: 12.85,13.63 JP2.1
  Route15 0.406: 11.91,11.35 v11.89,11.33 11.07,11.33 10.62,10.87 10.62,7.06 9.5,5.94 7.54,5.94 7.18,5.58 7.18,2.26 6.25,1.33 JP3.1
VLXSMPS
  Top 0.203: 7.2,32.68 L2.2
  Top 0.305: U1.P$33 7.25,32.49 L2.2

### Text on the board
tPlace: STM32WB55 | Firefly | 13 | 12 | SCL | 11 | SDA | 10 | A0 | 9 | A1 | 8 | 7 | A2 | A3 | 6 | A4 | 5 | 4 | CLK | - | + | DIO | 3 | 2 | nRST | 3V3 | 1 | nRST | BTN | 0 | GND | VIN | GND
bPlace: FireFly | Pesky Products | v.01b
